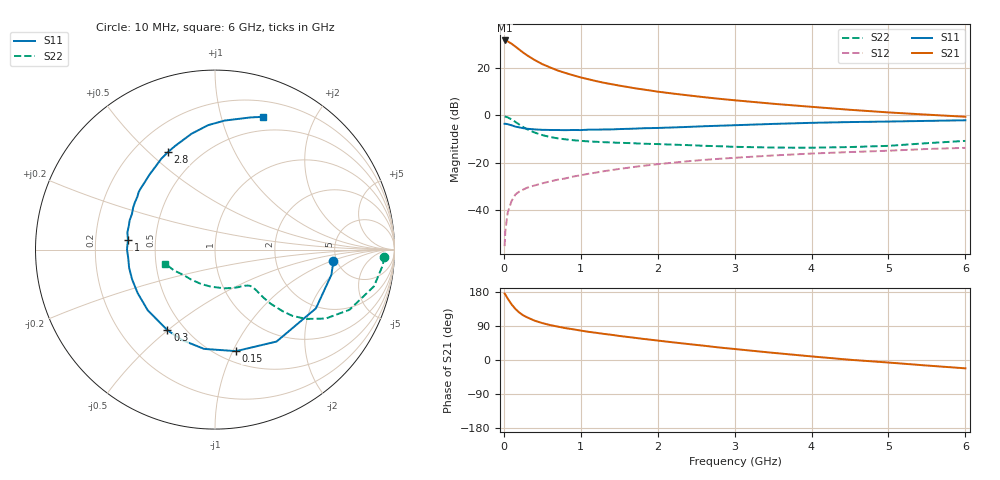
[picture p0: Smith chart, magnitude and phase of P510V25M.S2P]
! SIEMENS Small Signal Semiconductors
! BFP183
! Si NPN RF Bipolar Junction Transistor in SOT143
! VCE = 10 V  IC = 25 mA
! Common Emitter S-Parameters:  March  1996
# GHz  S  MA  R  50
!  f  S11  S21  S12  S22
! GHz  MAG  ANG  MAG  ANG  MAG  ANG  MAG  ANG
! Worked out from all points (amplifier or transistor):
!   36 points, 10 MHz to 6 GHz, reference 50 ohm
!   highest |S21| = 31.7 dB at 10 MHz (marker M1)
!   |S21| within 3 dB of that: start of sweep to 166.5 MHz
!   unconditionally stable (mu >= 1): 899.1 MHz to 5.934 GHz
!   at 250 MHz: K = 0.48, MSG = 29.0 dB, |S12| = -31.5 dB
!   at 1.4 GHz: K = 1.12, MAG = 16.1 dB, |S12| = -23.2 dB
!   at 6 GHz: K = 0.99, MSG = 6.6 dB, |S12| = -13.8 dB
!   S11 on the Smith chart (normalised r, x): 10 MHz: 4.67, -1.08; 150 MHz: 0.61, -1.03; 300 MHz: 0.40, -0.50; 1 GHz: 0.35, +0.05; 2.8 GHz: 0.34, +0.58; 6 GHz: 0.35, +1.37
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0.01  0.6628 -5.6  38.53 175.4  0.0017 69.1  0.9426 -2.4
0.02  0.6636 -12.2  38.13 172.5  0.0036 70.8  0.939 -5.3
0.05  0.6507 -30.2  36.9 162.1  0.0087 74.7  0.909 -13.0
0.1  0.6165 -56.2  32.88 147.0  0.0153 63.7  0.821 -24.1
0.15  0.5778 -78.3  28.61 134.8  0.0211 58.4  0.7268 -31.9
0.2  0.5565 -96.3  24.77 125.4  0.0243 53.8  0.639 -37.2
0.25  0.5365 -109.8  21.4 118.1  0.0267 50.7  0.5669 -40.6
0.3  0.5214 -120.6  18.77 112.8  0.0293 49.5  0.5103 -42.3
0.4  0.5046 -138.0  14.87 103.8  0.0328 48.8  0.4328 -44.2
0.5  0.4944 -150.6  12.16 97.4  0.0364 48.6  0.382 -44.7
0.6  0.4907 -160.3  10.38 92.3  0.0399 49.2  0.3485 -44.7
0.7  0.4892 -167.9  8.916 88.1  0.0435 50.6  0.3259 -44.6
0.8  0.4859 -175.1  7.901 84.2  0.0462 50.7  0.3105 -44.7
1  0.4879 173.8  6.351 77.6  0.0539 51.6  0.2884 -45.4
1.1  0.4975 168.9  5.807 74.4  0.058 51.8  0.2809 -46.0
1.5  0.5122 153.0  4.268 63.5  0.0734 51.3  0.2625 -50.0
2.2  0.5549 131.1  2.891 46.6  0.0997 46.8  0.2398 -62.2
2.8  0.6033 115.7  2.244 33.0  0.1203 41.5  0.222 -76.3
3.5  0.6589 101.4  1.761 18.9  0.1415 35.4  0.2079 -96.0
4.5  0.7211 85.7  1.312 0.6  0.1671 26.3  0.2134 -128.5
5.5  0.7633 74.8  1.036 -14.6  0.1941 18.9  0.2576 -153.5
6  0.7872 70.0  0.934 -22.0  0.2052 14.4  0.2882 -164.4
